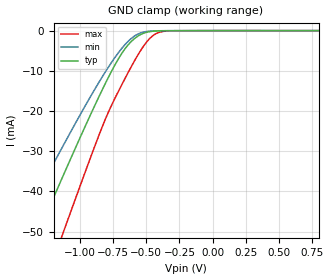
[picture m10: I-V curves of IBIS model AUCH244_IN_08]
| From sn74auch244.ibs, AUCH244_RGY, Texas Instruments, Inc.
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[Model]   AUCH244_IN_08
Model_type  Input
Vinl=0.28
Vinh=0.52
| variable   typ   min   max
C_comp   2.61pF   2.20pF   2.90pF
[Temperature Range]   40   100   -40
| Ambient temperature   25   85   -40
[Voltage range]   0.8   0.8   0.8
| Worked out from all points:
|   GND clamp passes 1 mA (typ) near -0.54 V on its own axis
[GND Clamp]
| AUCH244_IN_08
|   Voltage   I(typ)   I(min)   I(max)
-3.6V     -227.9mA   -191.3mA   -273.4mA
-1.49V    -63.73mA   -51.31mA   -83.4mA
-1.45V    -60.66mA   -48.76mA   -79.76mA
-1.31V    -49.93mA   -39.92mA   -66.98mA
-1.14V    -37.05mA   -29.4mA    -51.45mA
-1.105V   -34.43mA   -27.28mA   -48.25mA
-835mV    -14.91mA   -11.65mA   -24.16mA
-700mV    -6.466mA   -5.052mA   -14.45mA
-580mV    -1.765mA   -1.17mA    -7.006mA
-450mV    -155.5uA   -81.7uA    -1.262mA
-310mV    -21.8uA    -14.36uA   -51.94uA
800mV     101.9pA    187.8pA    82.48pA
